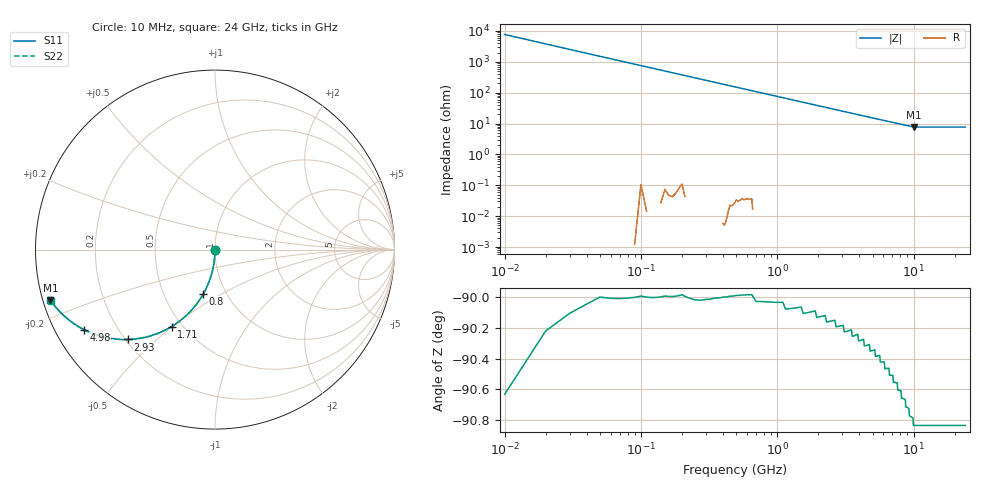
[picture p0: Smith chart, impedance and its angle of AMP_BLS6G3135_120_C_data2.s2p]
! Created Mon May 10 11:41:15 2010
# ghz S ma R 50
! 2 Port Network Data from SP1.SP block
! freq  magS11  angS11  magS21  angS21  magS12  angS12  magS22  angS22
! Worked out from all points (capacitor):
!   2400 points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, 10 MHz to 24 GHz, reference 50 ohm
!   read as one part in shunt: C = 2.1 pF near 130 MHz
!   lowest |Z| = 7.7 ohm at 10 GHz (marker M1)
!   S11 on the Smith chart (normalised r, x): 10 MHz: 1.00, -0.01; 800 MHz: 0.78, -0.41; 1.71 GHz: 0.44, -0.50; 2.93 GHz: 0.21, -0.41; 4.98 GHz: 0.08, -0.28; 24 GHz: 0.02, -0.15
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0.01  0.003216 -89.6  1 -0.2  1 -0.2  0.003264 -89.3
0.07  0.02294 -91.3  0.9997 -1.3  0.9997 -1.3  0.02316 -91.3
0.15  0.04907 -92.8  0.9988 -2.8  0.9988 -2.8  0.04955 -92.8
0.19  0.06215 -93.6  0.998 -3.6  0.998 -3.6  0.06276 -93.6
0.25  0.08309 -94.7  0.9966 -4.7  0.9966 -4.7  0.08233 -94.7
0.35  0.1154 -96.6  0.9933 -6.6  0.9933 -6.6  0.115 -96.6
0.47  0.1537 -98.8  0.988 -8.9  0.988 -8.9  0.1537 -98.8
0.62  0.2005 -101.6  0.9795 -11.6  0.9795 -11.6  0.201 -101.6
0.8  0.2562 -104.8  0.9667 -14.8  0.9667 -14.8  0.2559 -104.8
1.2  0.3694 -111.6  0.9297 -21.7  0.9297 -21.7  0.3689 -111.6
1.71  0.4925 -119.4  0.871 -29.5  0.871 -29.5  0.4923 -119.4
2.3  0.6063 -127.1  0.7969 -37.3  0.7969 -37.3  0.6054 -127.1
2.93  0.6962 -134.0  0.7197 -44.2  0.7197 -44.2  0.696 -133.9
4.01  0.7994 -142.9  0.6043 -53.1  0.6043 -53.1  0.7989 -142.8
4.98  0.8557 -148.6  0.5219 -58.9  0.5219 -58.9  0.8554 -148.5
6.34  0.9037 -154.4  0.4343 -64.8  0.4343 -64.8  0.9035 -154.2
8.01  0.9367 -159.2  0.358 -69.7  0.358 -69.7  0.9368 -159.0
10  0.9588 -163.0  0.2952 -73.7  0.2952 -73.7  0.9589 -162.8
12.01  0.9588 -163.0  0.2952 -73.7  0.2952 -73.7  0.9589 -162.8
16.01  0.9588 -163.0  0.2952 -73.7  0.2952 -73.7  0.9589 -162.8
20.01  0.9588 -163.0  0.2952 -73.7  0.2952 -73.7  0.9589 -162.8
24  0.9588 -163.0  0.2952 -73.7  0.2952 -73.7  0.9589 -162.8
